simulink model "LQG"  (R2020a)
settings: Solver=VariableStepAuto  StartTime=0.0  StopTime=10.0  RelTol=1e-3
PreLoadFcn:
  | initParams
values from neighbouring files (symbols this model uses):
  A = [-2 -2 1;0 -2 -1;0 0 -2]    [initParams.m]
  B = [0 1 1;0 0 2;1 0 0]    [initParams.m]
  C = [1 0]    [initParams.m]
  K = 10    [initParams.m]
  L = place(A',C',ev).'    [initParams.m]
  V = 0.1    [initParams.m]
  W = [0.1 0;0 0.1]    [initParams.m]
  x0 = [0.2;0.1]    [initParams.m]
  x0s = [0;0]    [initParams.m]
undefined symbols (not defined in the file or in its folder): Continuous, Time
libraries: ctrlSharedLib x1

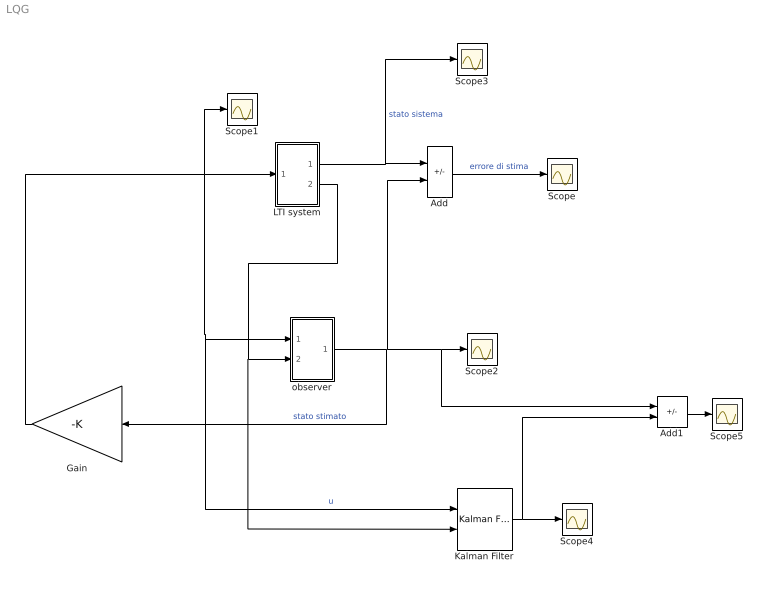
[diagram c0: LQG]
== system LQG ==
  Add : Sum  Inputs=+-
  Add1 : Sum  Inputs=+-
  Gain : Gain  Gain=-K  Multiplication=Matrix(K*u) (u vector)
  Kalman Filter : ctrlSharedLib/Kalman Filter  TimeDomain=Continuous-Time  UseCurrentEstimator=on  ModelSource=Individual A, B, C, D matrices  ModelSourceVariable=ss(0.95,1,1,0,1)  A=A  B=B  C=C  D=0  NumberOfStates=1  NumberOfInputs=1  NumberOfOutputs=1  InitialEstimateSource=Dialog  X0=x0s  P0=10  UseK=off  UseGH=off  NumberOfProcessNoiseInputs=1  G=1  TimeInvariantG=on  H=0  TimeInvariantH=on  Q=W  TimeInvariantQ=on  R=V  TimeInvariantR=on  N=0  TimeInvariantN=on  AddInputPort=on  AddEnablePort=off  OutputEstimatedY=off  OutputP=off  Ts=-1
  LTI system : Subsystem
  Scope{,1..5} (6 alike) : Scope
  observer : Subsystem
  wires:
  LTI system/2(y) -> Kalman Filter/2, observer/2(y)
  Gain/1 -> Kalman Filter/1, observer/1(u), Scope1/1, LTI system/1(u)  "u"
  LTI system/1(x) -> Scope3/1, Add/1  "stato sistema"
  observer/1(xHat) -> Add/2, Add1/1, Scope2/1, Gain/1  "stato stimato"
  Add/1 -> Scope/1  "errore di stima"
  Kalman Filter/1 -> Add1/2, Scope4/1
  Add1/1 -> Scope5/1

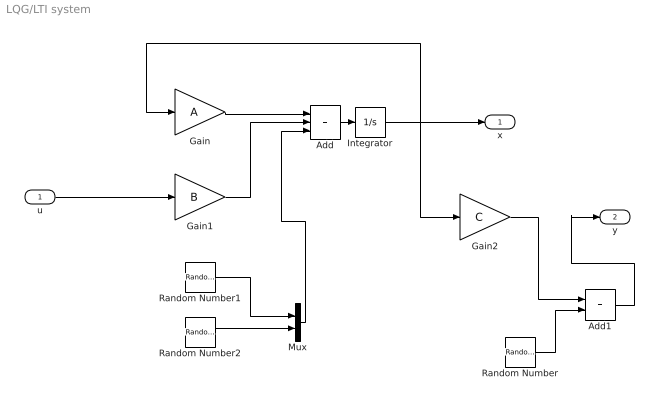
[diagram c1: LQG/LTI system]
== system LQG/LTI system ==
  u : Inport
  Add : Sum  Inputs=+++
  Add1 : Sum
  Gain : Gain  Gain=A  Multiplication=Matrix(K*u) (u vector)
  Gain1 : Gain  Gain=B  Multiplication=Matrix(K*u) (u vector)
  Gain2 : Gain  Gain=C  Multiplication=Matrix(K*u) (u vector)
  Integrator : Integrator  InitialCondition=x0
  Mux : Mux  Inputs=2
  Random Number : RandomNumber  Variance=V  SampleTime=0.01
  Random Number1 : RandomNumber  Variance=W(1,1)  SampleTime=0.01
  Random Number2 : RandomNumber  Variance=W(2,2)  SampleTime=0.01
  x : Outport
  y : Outport  Port=2
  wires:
  Gain1/1 -> Add/2
  Integrator/1 -> x/1, Gain2/1, Gain/1
  Gain/1 -> Add/1
  Add/1 -> Integrator/1
  u/1 -> Gain1/1
  Random Number/1 -> Add1/2
  Add1/1 -> y/1
  Gain2/1 -> Add1/1
  Random Number1/1 -> Mux/1
  Random Number2/1 -> Mux/2
  Mux/1 -> Add/3

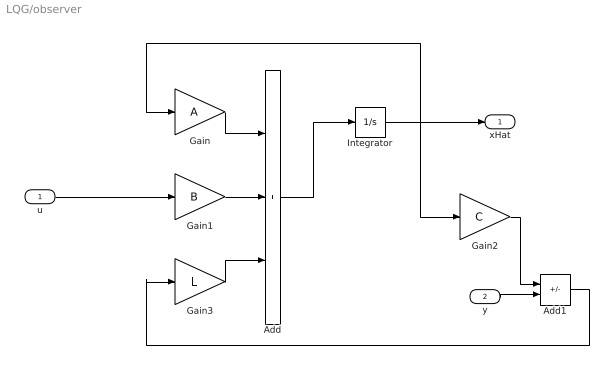
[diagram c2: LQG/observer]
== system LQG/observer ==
  u : Inport
  y : Inport  Port=2
  Add : Sum  Inputs=+++
  Add1 : Sum  Inputs=-+
  Gain : Gain  Gain=A  Multiplication=Matrix(K*u) (u vector)
  Gain1 : Gain  Gain=B  Multiplication=Matrix(K*u) (u vector)
  Gain2 : Gain  Gain=C  Multiplication=Matrix(K*u) (u vector)
  Gain3 : Gain  Gain=L  Multiplication=Matrix(K*u) (u vector)
  Integrator : Integrator  InitialCondition=x0s
  xHat : Outport
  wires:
  Gain1/1 -> Add/2
  Integrator/1 -> xHat/1, Gain2/1, Gain/1
  Gain/1 -> Add/1
  Add/1 -> Integrator/1
  u/1 -> Gain1/1
  Gain2/1 -> Add1/1
  y/1 -> Add1/2
  Gain3/1 -> Add/3
  Add1/1 -> Gain3/1
